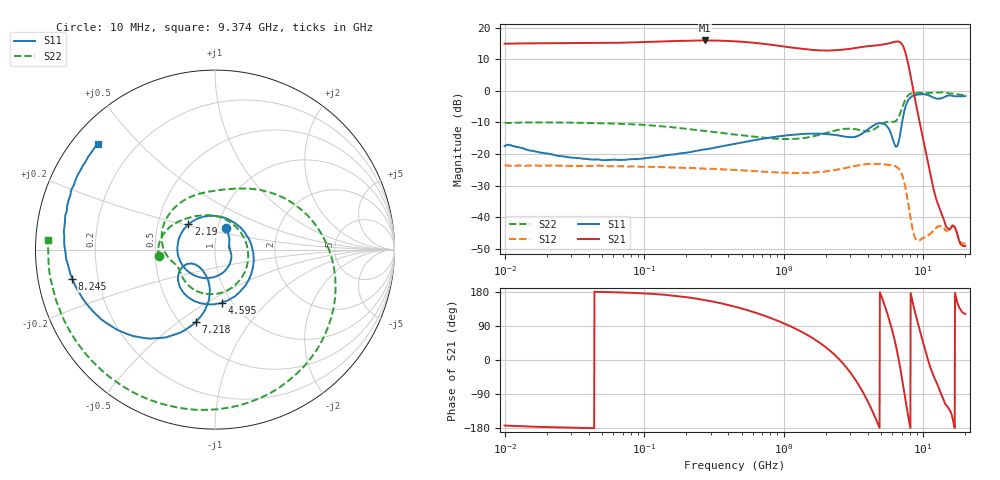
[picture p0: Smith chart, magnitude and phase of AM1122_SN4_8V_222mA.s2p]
!Agilent Technologies,E8364B,MY43040894,A.07.50.67
!Agilent E8364B: A.07.50.67
!Date: Thursday, July 29, 2021 08:03:52
!Correction: S11(Full 2 Port(1,2))
!S21(Full 2 Port(1,2))
!S12(Full 2 Port(1,2))
!S22(Full 2 Port(1,2))
!S2P File: Measurements: S11, S21, S12, S22:Log Frequency Sweep
# Hz S  dB  R 50
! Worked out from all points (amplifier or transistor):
!   1601 points, 10 MHz to 20.05 GHz, reference 50 ohm
!   highest |S21| = 16.0 dB at 273.2 MHz (marker M1)
!   |S21| within 3 dB of that: 2.549 GHz to 7.351 GHz (4.801 GHz wide, 97 % of centre)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
!   unconditionally stable (mu >= 1): start of sweep to end of sweep
!   at 35.4 MHz: K = 1.38, MAG = 15.8 dB, |S12| = -23.8 dB
!   at 447.8 MHz: K = 1.55, MAG = 16.0 dB, |S12| = -25.1 dB
!   at 20.05 GHz: K = 3254.23, MAG = -38.6 dB, |S12| = -48.2 dB
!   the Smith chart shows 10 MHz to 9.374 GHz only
!   S11 on the Smith chart (normalised r, x): 10 MHz: 1.10, +0.26; 2.19 GHz: 0.72, +0.21; 4.595 GHz: 0.90, -0.59; 7.218 GHz: 0.60, -0.58; 8.245 GHz: 0.11, -0.10; 9.374 GHz: 0.07, +0.38
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1e7  -17.50 62.5  14.93 -173.1  -23.60 3.0  -10.09 -173.3
3.556644e7  -21.43 20.0  15.11 -179.3  -23.78 -1.6  -10.12 173.0
1.264971e8  -20.84 -12.7  15.61 173.4  -24.12 -10.5  -11.14 151.8
2.731617e8  -18.51 -49.2  15.96 158.1  -24.65 -19.6  -12.73 130.6
4.499052e8  -16.76 -82.8  15.69 140.4  -25.07 -29.2  -13.85 109.3
8.834534e8  -14.52 -133.4  14.39 105.1  -25.83 -49.5  -15.18 60.6
1.592566e9  -13.54 175.8  12.97 59.0  -25.89 -80.2  -14.51 -10.5
2.189644e9  -13.79 136.4  12.78 21.8  -25.24 -109.1  -12.91 -59.5
2.925948e9  -14.66 74.9  13.25 -27.5  -24.21 -150.9  -11.95 -109.1
3.65819e9  -13.53 -1.8  13.90 -82.0  -23.38 161.5  -12.61 -143.5
4.595468e9  -10.51 -82.3  14.39 -157.1  -23.17 95.1  -11.78 -168.3
5.126224e9  -10.29 -117.2  14.64 158.5  -23.25 56.8  -10.32 167.2
5.664191e9  -12.02 -144.9  15.03 110.0  -23.45 15.5  -9.78 133.5
6.111657e9  -15.86 -150.9  15.43 66.1  -23.66 -21.9  -9.82 102.6
6.56321e9  -17.11 -116.8  15.64 15.0  -24.34 -64.6  -8.86 70.6
6.850002e9  -13.45 -98.0  15.35 -22.1  -25.37 -95.0  -7.05 45.5
7.217599e9  -7.63 -104.7  13.88 -72.8  -27.99 -136.4  -4.19 4.2
7.677546e9  -3.54 -133.7  9.91 -134.0  -33.67 179.4  -1.75 -52.6
8.244793e9  -1.82 -168.5  3.15 165.8  -42.01 153.0  -0.82 -110.3
9.373525e9  -1.12 137.8  -9.41 83.0  -47.41 139.0  -0.62 176.7
1.417279e10  -1.98 -47.5  -41.28 -111.3  -43.62 -82.2  -0.54 5.2
2.005e10  -1.69 -174.8  -49.17 121.3  -48.18 127.4  -1.39 -135.9
